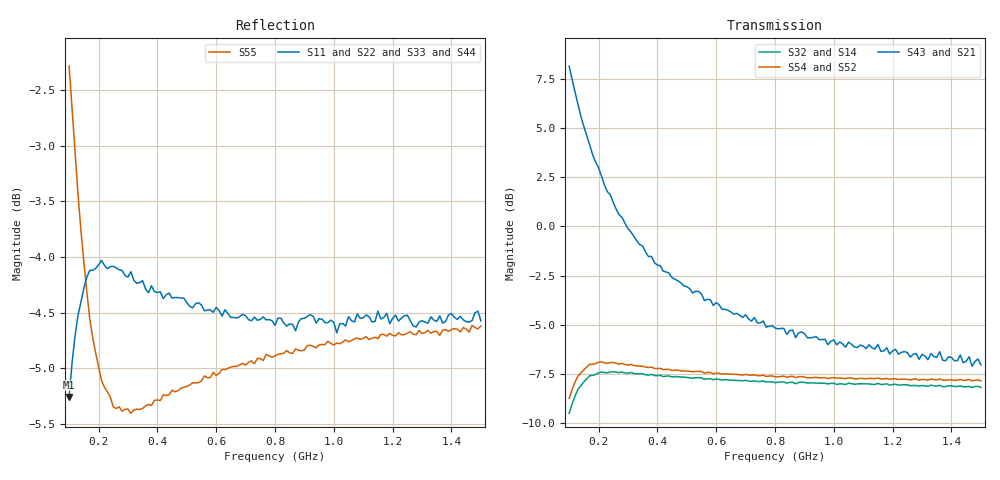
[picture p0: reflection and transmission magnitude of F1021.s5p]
!  POLYFET RF DEVICES
!  F1021
!  S PARAMETERS
!  VDS=28V, IDQ=800mA
! Date: Mon Oct 21 18:10:46 1991
! Bias (V mA) : V1=2.5299000  I1=0.0051051  V2=27.993660  I2=702.49320
!AWR Design Environment (2053) Wed Feb 04 14:41:54 2004
!freq-unit  param-type  data-format  keyword  impedance-ohms
# MHz  S  MA  R  50
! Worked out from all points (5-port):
!   141 points, 100 MHz to 1.5 GHz, reference 50 ohm
!   strongest paths, dB at 100 MHz, 450 MHz, 800 MHz, 1.15 GHz, 1.5 GHz:
!     S43: 8.1, -2.6, -5.1, -6.0, -7.0
!     S21: 8.1, -2.6, -5.1, -6.0, -7.0
!     S54: -8.7, -7.3, -7.6, -7.7, -7.8
!     S52: -8.7, -7.3, -7.6, -7.7, -7.8
!     S32: -9.5, -7.6, -7.9, -8.0, -8.2
!     S14: -9.5, -7.6, -7.9, -8.0, -8.2
!   lowest |S11| = -5.3 dB at 100 MHz (marker M1), VSWR 3.41, Z = 19.4 - j26.8 ohm
!   |S11| at or under -10 dB: nowhere
